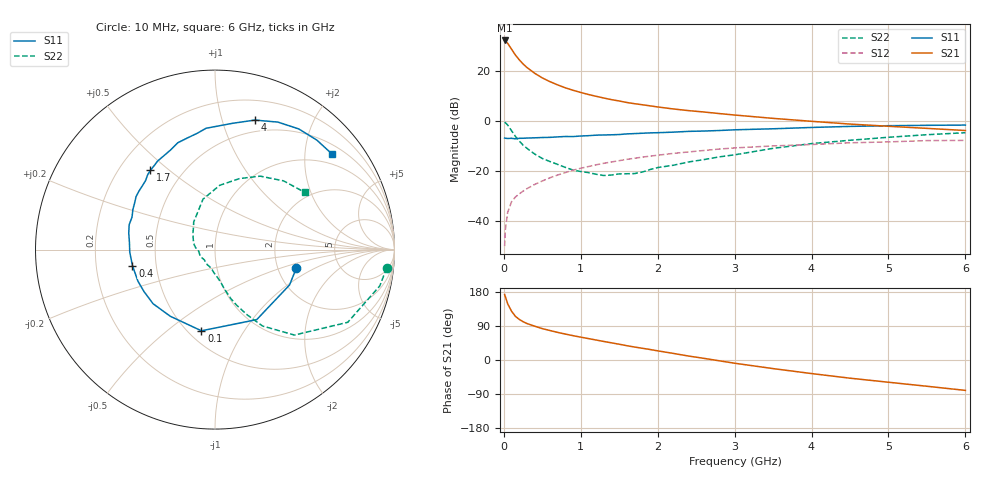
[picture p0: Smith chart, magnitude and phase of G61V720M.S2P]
! SIEMENS Small Signal Semiconductors
! BFG193
! Si NPN RF Bipolar Junction Transistor in SOT223
! VCE = 1.75 V  IC = 20 mA
! Common Emitter S-Parameters:  August  1996
# GHz  S  MA  R  50
!  f  S11  S21  S12  S22
! GHz  MAG  ANG  MAG  ANG  MAG  ANG  MAG  ANG
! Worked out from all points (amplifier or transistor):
!   36 points, 10 MHz to 6 GHz, reference 50 ohm
!   highest |S21| = 32.3 dB at 10 MHz (marker M1)
!   |S21| within 3 dB of that: start of sweep to 89.62 MHz
!   unconditionally stable (mu >= 1): 649.7 MHz to 2.694 GHz
!   at 250 MHz: K = 0.75, MSG = 25.4 dB, |S12| = -27.9 dB
!   at 1.4 GHz: K = 1.06, MAG = 11.0 dB, |S12| = -16.2 dB
!   at 6 GHz: K = 0.92, MSG = 2.0 dB, |S12| = -7.6 dB
!   S11 on the Smith chart (normalised r, x): 10 MHz: 2.53, -0.66; 100 MHz: 0.58, -0.66; 400 MHz: 0.36, -0.08; 1.7 GHz: 0.33, +0.43; 4 GHz: 0.38, +1.28; 6 GHz: 0.73, +2.65
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0.01  0.4647 -12.8  41.39 172.9  0.0032 89.6  0.9621 -6.1
0.02  0.4598 -25.4  40.48 166.9  0.0069 81.2  0.9402 -12.4
0.05  0.4541 -59.2  36.21 148.3  0.0152 70.1  0.8434 -28.7
0.1  0.4587 -99.5  27.72 128.8  0.0247 60.4  0.65 -47.1
0.15  0.4473 -123.9  21.18 115.3  0.0307 55.9  0.5016 -58.1
0.2  0.4582 -138.8  17.02 107.2  0.0355 56.5  0.4064 -63.7
0.25  0.4596 -149.5  14.04 101.1  0.0403 56.2  0.3342 -68.6
0.3  0.464 -157.7  11.94 96.3  0.0451 57.0  0.2899 -71.9
0.4  0.4686 -169.1  9.162 89.3  0.0547 58.4  0.2227 -76.8
0.5  0.4751 -178.2  7.383 82.8  0.0643 58.3  0.1813 -80.5
0.6  0.4788 174.9  6.207 77.8  0.0745 58.6  0.1572 -84.6
0.7  0.4892 169.2  5.35 72.8  0.0847 58.0  0.1378 -89.9
0.9  0.4963 158.7  4.18 64.2  0.1057 55.7  0.1063 -100.7
1.1  0.5174 150.0  3.44 56.5  0.125 52.9  0.0945 -117.0
1.4  0.5387 138.7  2.715 45.3  0.1542 47.2  0.0847 -145.3
1.7  0.5696 129.2  2.251 34.2  0.183 41.4  0.0904 -172.9
2.2  0.6081 113.9  1.771 17.5  0.2285 30.0  0.1323 156.0
3.5  0.7103 82.1  1.147 -22.7  0.3228 -0.8  0.2887 103.4
4  0.755 72.9  1.002 -35.8  0.3443 -10.5  0.3593 85.8
4.5  0.7923 63.7  0.882 -48.0  0.3725 -20.5  0.4189 70.9
5.5  0.8331 47.1  0.724 -69.3  0.4125 -43.3  0.5408 45.1
6  0.8423 39.0  0.656 -80.2  0.416 -56.5  0.5927 32.6
